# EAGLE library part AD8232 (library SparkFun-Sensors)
AD8232 Single Lead Heart Rate Monitor IC Datasheet SparkFun Products SparkFun Single Lead Heart Rate Monitor - AD8232 (SEN-12650)
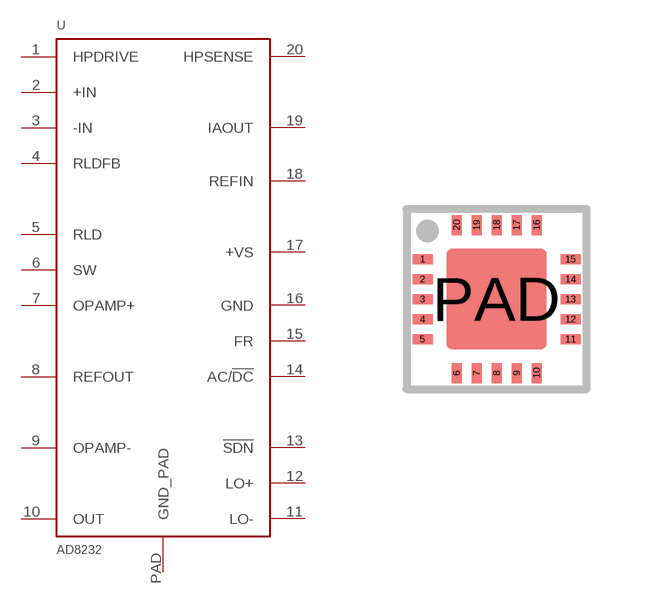
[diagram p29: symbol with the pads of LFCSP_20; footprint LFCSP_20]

Designator prefix -

## AD8232 (PROD_ID: IC-11886; VALUE: AD8232ACPZ-R7)  [LFCSP_20]
1  HPDRIVE
2  +IN
3  -IN
4  RLDFB
5  RLD
6  SW
7  OPAMP+
8  REFOUT
9  OPAMP-
10  OUT
11  LO-
12  LO+
13  !SDN
14  AC/!DC
15  FR
16  GND
17  +VS
18  REFIN
19  IAOUT
20  HPSENSE
PAD  GND_PAD

## Footprint LFCSP_20 (pad centres in mm)
smd 0.5 x 0.25: 1 -1.85,1; 2 -1.85,0.5; 3 -1.85,0; 4 -1.85,-0.5; 5 -1.85,-1; 11 1.85,-1; 12 1.85,-0.5; 13 1.85,0; 14 1.85,0.5; 15 1.85,1
smd 0.25 x 0.5: 6 -1,-1.85; 7 -0.5,-1.85; 8 0,-1.85; 9 0.5,-1.85; 10 1,-1.85; 16 1,1.85; 17 0.5,1.85; 18 0,1.85; 19 -0.5,1.85; 20 -1,1.85
smd 2.5 x 2.5: PAD 0,0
